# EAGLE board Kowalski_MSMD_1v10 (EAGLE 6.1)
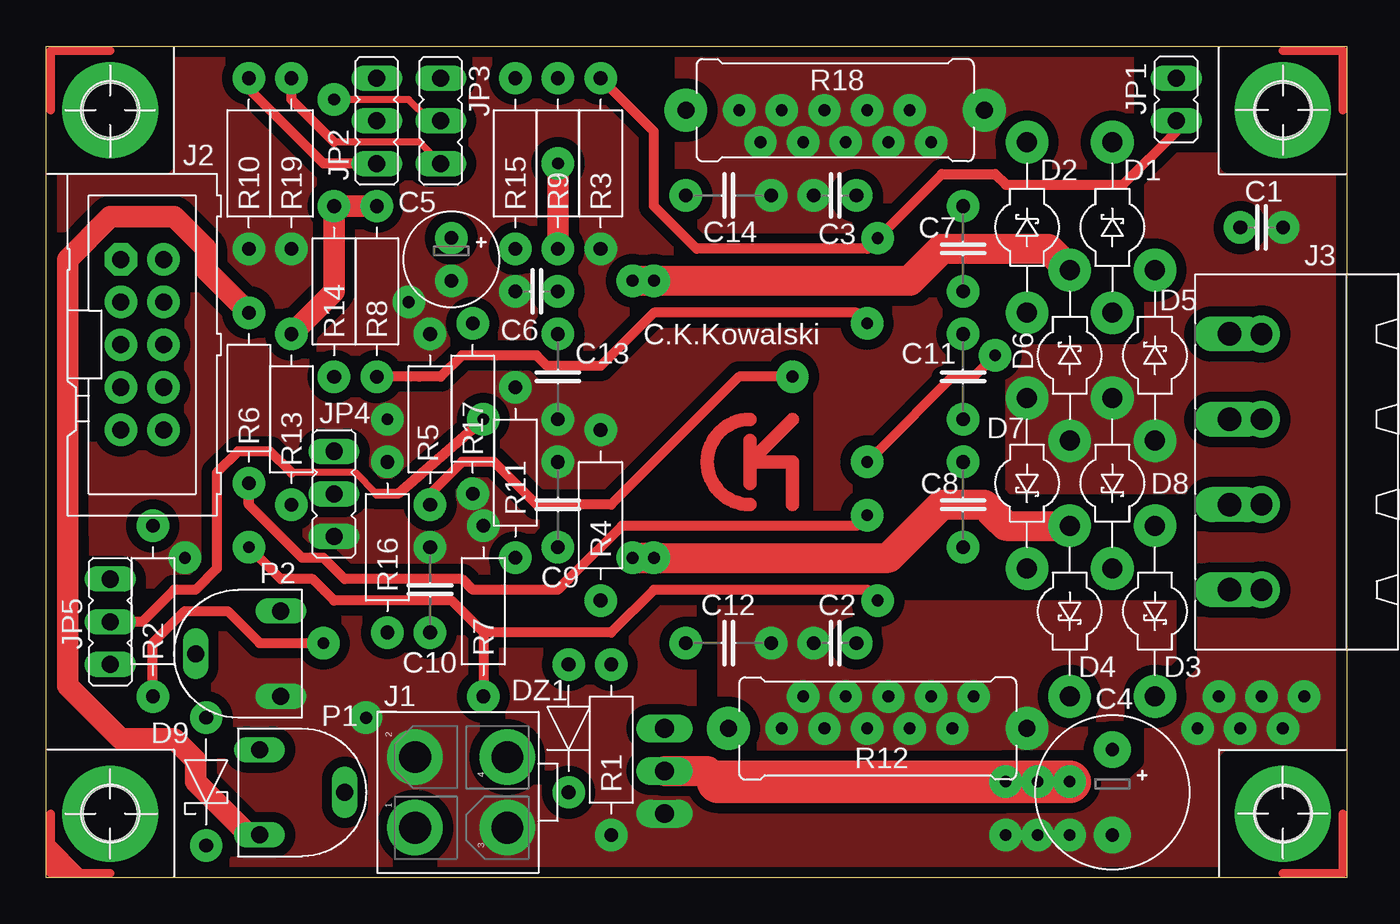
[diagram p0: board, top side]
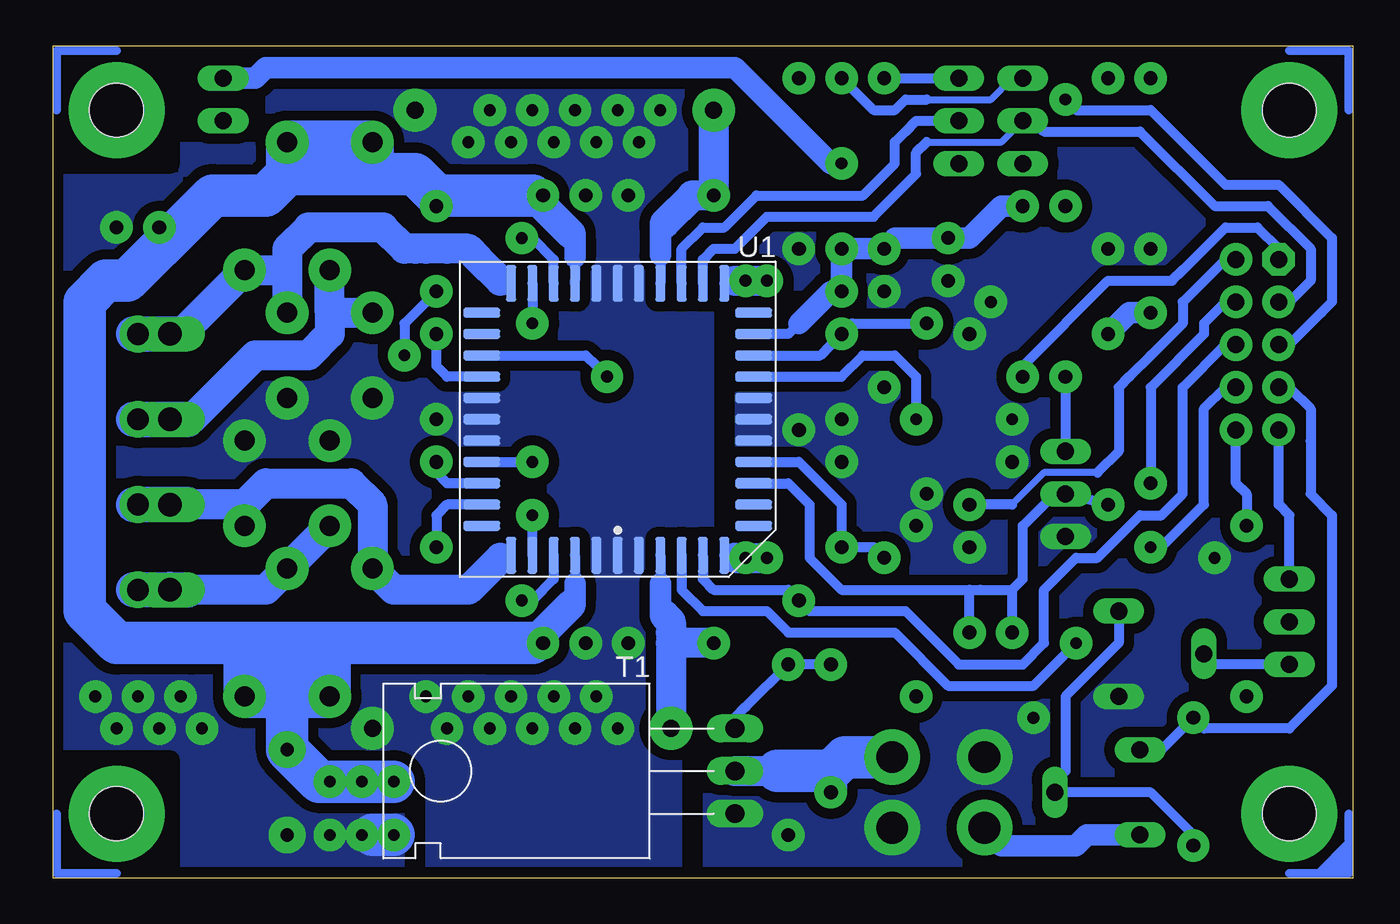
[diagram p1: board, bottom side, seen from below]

Size 77.47 x 49.53 mm. Coordinates in mm from the lower left corner, seen from the top.
Outline: 0,0 0,49.53 77.47,49.53 77.47,0 0,0
Copper layers (1*16): Top 0.035mm / dielectric 1.5mm / Bottom 0.035mm
Design rules: minimum track width 32mil, minimum drill 24mil, track to track 8mil, track to pad 8mil, pad to pad 8mil, via to via 8mil, smd to smd 8mil, copper to edge 25mil, drill to drill 8mil, minimum pad ring 10mil, minimum via ring 8mil, stop-mask expansion 4mil, vias tented up to drill 0mil, thermal gap 12mil
tRestrict: area 53.3,23.5 to 56.5,29.8; area 39.4,21.6 to 45.1,27.9; area 44.5,27.9 to 45.1,29.2; 21 lines
bRestrict: 6 lines

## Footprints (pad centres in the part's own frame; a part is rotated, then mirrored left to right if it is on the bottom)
C2.5 = drill 0.813 pad 1.93: 1 -1.27,0; 2 1.27,0
CE5 = drill 0.8 pad 2.184: + -2.54,0; - 2.54,0
CE2.5 = drill 0.8 pad 1.93: + -1.27,0; - 1.27,0
C5 = drill 0.813 pad 1.93: 1 -2.54,0; 2 2.54,0
DS = drill 1.194 pad 2.54: A 5.08,0; C -5.08,0
DS7,5 = drill 0.813 pad 1.93: A 3.81,0; C -3.81,0
DZ7,5 = drill 0.813 pad 1.93: A 3.81,0; C -3.81,0
MF-04-V = drill 1.9 pad 3.3: 1 2.1,-2.8; 2 -2.1,-2.8; 3 2.1,2.7; 4 -2.1,2.7
ML10 = drill 1.016 pad 1.93 octagon: 1 -5.08,-1.27 | drill 1.016 pad 1.93: 2 -5.08,1.27; 3 -2.54,-1.27; 4 -2.54,1.27; 5 0,-1.27; 6 0,1.27; 7 2.54,-1.27; 8 2.54,1.27; 9 5.08,-1.27; 10 5.08,1.27
MSTBA4 = drill 1.397 long: 1 -7.62,5.08; 2 -2.54,5.08; 3 2.54,5.08; 4 7.62,5.08
JP1 = drill 1.016 pad 1.422 long: 1 0,-1.27; 2 0,1.27
JP2 = drill 1.016 pad 1.422 long: 1 -2.54,0; 2 0,0; 3 2.54,0
CA6V = drill 1.016 long: A -2.54,-2.54; E 2.54,-2.54; S 0,2.54
0309/10 = drill 0.813 pad 1.93: 1 -5.08,0; 2 5.08,0
0617/17 = drill 1.016 pad 2.54: 1 -8.89,0; 2 8.89,0
TO220AH = drill 1.118 long: B 2.54,-6.35; C 0,-6.35; E -2.54,-6.35
STEPPER_PLCC44 = smd 0.6 x 2.2: 1 0,8.1; 2 -1.27,8.1; 3 -2.54,8.1; 4 -3.81,8.1; 5 -5.08,8.1; 6 -6.35,8.1; 18 -6.35,-8.1; 19 -5.08,-8.1; 20 -3.81,-8.1; 21 -2.54,-8.1; 22 -1.27,-8.1; 23 0,-8.1; 24 1.27,-8.1; 25 2.54,-8.1; 26 3.81,-8.1; 27 5.08,-8.1; 28 6.35,-8.1; 40 6.35,8.1; 41 5.08,8.1; 42 3.81,8.1; 43 2.54,8.1; 44 1.27,8.1 | smd 2.2 x 0.6: 7 -8.1,6.35; 8 -8.1,5.08; 9 -8.1,3.81; 10 -8.1,2.54; 11 -8.1,1.27; 12 -8.1,0; 13 -8.1,-1.27; 14 -8.1,-2.54; 15 -8.1,-3.81; 16 -8.1,-5.08; 17 -8.1,-6.35; 29 8.1,-6.35; 30 8.1,-5.08; 31 8.1,-3.81; 32 8.1,-2.54; 33 8.1,-1.27; 34 8.1,0; 35 8.1,1.27; 36 8.1,2.54; 37 8.1,3.81; 38 8.1,5.08; 39 8.1,6.35
CORNER_HOLE_3.2MM = hole 3.2: 0,0
CORNER_HOLE_3.2MM_SIGN = hole 3.2: 0,0

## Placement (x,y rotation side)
C1  100n  [C2.5]  72.39,38.73 0 top
C2  100n  [C2.5]  46.99,13.97 180 top
C3  3x100n  [C2.5]  46.99,40.64 180 top
C4  470u  [CE5]  63.5,5.08 270 top
C5  100u  [CE2.5]  24.13,36.83 270 top
C6  100n  [C2.5]  29.21,34.92 180 top
C7  220n  [C5]  54.61,37.47 270 top
C8  220n  [C5]  54.61,22.23 270 top
C9  1n  [C5]  30.48,22.23 90 top
C10  100n  [C5]  22.86,17.14 90 top
C11  220n  [C5]  54.61,29.84 270 top
C12  100n  [C5]  40.64,13.97 0 top
C13  1n  [C5]  30.48,29.84 90 top
C14  100n  [C5]  40.64,40.64 0 top
D1  DS  [DS]  63.5,38.73 270 top
D2  DS  [DS]  58.42,38.73 270 top
D3  8xBYV27  [DS]  66.04,15.88 90 top
D4  DS  [DS]  60.96,15.88 90 top
D5  DS  [DS]  66.04,31.11 270 top
D6  DS  [DS]  60.96,31.11 270 top
D7  DS  [DS]  58.42,23.5 90 top
D8  DS  [DS]  63.5,23.5 90 top
D9  BAT85  [DS7,5]  9.53,5.71 90 top
DZ1  30V  [DZ7,5]  31.11,8.89 90 top
J1  MF-04  [MF-04-V]  24.77,5.08 270 top
J2  ML10  [ML10]  5.71,31.75 270 top
J3  MSTBA4  [MSTBA4]  75.56,24.77 90 top
JP1  [JP1]  67.31,46.35 180 top
JP2  [JP2]  19.68,45.09 270 top
JP3  [JP2]  23.5,45.09 270 top
JP4  [JP2]  17.14,22.86 270 top
JP5  [JP2]  3.81,15.24 90 top
P1  4k7  [CA6V]  15.24,5.08 270 top
P2  4k7  [CA6V]  11.43,13.34 90 top
R1  4k7  [0309/10]  33.66,7.62 270 top
R2  4k7  [0309/10]  6.35,15.88 270 top
R3  4k7  [0309/10]  33.02,42.55 90 top
R4  4k7  [0309/10]  33.02,21.59 270 top
R5  4k7  [0309/10]  22.86,27.3 270 top
R6  15k  [0309/10]  12.06,28.57 270 top
R7  15k  [0309/10]  26.04,15.88 270 top
R8  15k  [0309/10]  19.68,34.92 270 top
R9  4k7  [0309/10]  30.48,42.55 90 top
R10  4k7  [0309/10]  12.06,42.55 90 top
R11  47k  [0309/10]  27.94,24.13 270 top
R12  0R22  [0617/17]  49.53,8.89 180 top
R13  10k  [0309/10]  14.61,27.3 90 top
R14  4k7  [0309/10]  17.14,34.92 270 top
R15  4k7  [0309/10]  27.94,42.55 90 top
R16  1k  [0309/10]  20.32,19.68 270 top
R17  47k  [0309/10]  25.4,27.94 90 top
R18  0R22  [0617/17]  46.99,45.72 180 top
R19  4k7  [0309/10]  14.61,42.55 90 top
T1  TIP130  [TO220AH]  43.18,6.35 90 bottom
U1  A3977  [STEPPER_PLCC44]  43.81,27.3 180 bottom
U$7  [CORNER_HOLE_3.2MM]  73.66,3.81 180 top
U$8  [CORNER_HOLE_3.2MM]  3.81,45.72 0 top
U$9  [CORNER_HOLE_3.2MM]  73.66,45.72 270 top
U$10  [CORNER_HOLE_3.2MM_SIGN]  3.81,3.81 90 top

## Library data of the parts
C1-C14 D1-D9 R1-R11 R13-R17 R19 U$7-U$10 = Std
DZ1 J1 R12 R18 = STANDARD_CK
J2 = con-ml; OC_FARNELL: unknown; OC_NEWARK: unknown
J3 = con-phoenix-508; MF: FARNELL; MPN: 1757268; OC_FARNELL: 3705195; OC_NEWARK: 71C4163
JP1-JP5 = jumper
P1 P2 = pot
T1 = MSMD_1v4
U1 = MSMD_1v1

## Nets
+5V: C5.+ C6.1 J1.1 JP1.1 P1.E R6.1 R8.1 R9.1 R13.2 R14.1 R15.1 U1.16
\!ENABLE: J2.4 R6.2 U1.41
\!HOME: R2.2 U1.4
\!HOME1: J2.10 R2.1
\!RESET: J2.1 R8.2 U1.27
\!SLEEP: J2.8 R7.2 U1.42
BOOST: D9.A J2.7 P1.A
CP1: C8.1 U1.37
CP2: C8.2 U1.38
DIR: J2.6 R4.2 U1.5
EXVREF: J2.9 JP5.3
GND: C1.2 C2.2 C3.2 C4.- C5.- C6.2 C9.2 C10.2 C11.2 C12.2 C13.1 C14.2 D5.A D6.A D7.A D8.A J1.2 J1.3 JP4.3 P2.A R1.2 R3.1 R4.1 R5.1 R7.1 R10.1 R11.1 R12.1 R16.1 R17.1 R18.1 R19.1 T1.E U1.1 U1.2 U1.11 U1.12 U1.13 U1.22 U1.23 U1.24 U1.33 U1.34 U1.35 U1.44
MS1: J2.5 JP3.2 U1.20
MS2: J2.3 JP2.2 U1.19
N$3: D9.C P1.S P2.E
N$4: C12.1 R12.2 U1.3
N$5: JP5.1 P2.S
N$6: JP2.1 R9.2
N$8: C14.1 R18.2 U1.21
N$9: JP4.1 R14.2
N$10: JP2.3 R10.2
N$12: JP3.3 R19.2
N$13: JP3.1 R15.2
N$14: DZ1.A R1.1 T1.B
OUT1A: D4.A D8.C J3.1 U1.6
OUT1B: D3.A D7.C J3.2 U1.40
OUT2A: D2.A D6.C J3.3 U1.18
OUT2B: D1.A D5.C J3.4 U1.28
PFD: C10.1 JP4.2 R13.1 R16.2 U1.9
RC1: C9.1 R11.2 U1.10
RC2: C13.2 R17.2 U1.15
SR: JP1.2 R3.2 U1.26
STEP: J2.2 R5.2 U1.31
VCC: C1.1 C2.1 C3.1 C4.+ C7.1 D1.C D2.C D3.C D4.C DZ1.C J1.4 T1.C U1.25 U1.43
VCP: C7.2 U1.36
VREF: JP5.2 U1.14
VREG: C11.1 U1.32

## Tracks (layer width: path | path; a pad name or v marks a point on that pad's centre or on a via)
+5V  (via drill 0.7 pad 1.93)
  Top 1.27: R8.1 R14.1 17.14,34.92 R13.2 | R6.1 9.53,36.2 9.53,37.47 7.62,39.37 3.81,39.37 1.27,36.83 1.27,20.32 1.27,11.43 3.17,9.53 4.45,8.26 7.62,8.26 8.89,6.99 8.89,5.71 12.06,2.54 P1.E | v30.48,42.55 30.48,41.91 R9.1
  Bottom 0.61: U1.16 33.66,32.38 33.02,33.02
  Bottom 1.27: R8.1 20.95,40.01 22.86,38.1 C5.+ 27.3,38.1 R15.1 R9.1 C6.1 31.11,34.92 33.02,33.02 | R6.1 13.34,33.66 R13.2 | JP1.1 65.41,47.62 64.77,48.26 36.83,48.26 34.29,45.72 31.11,42.55 v30.48,42.55 | J1.1 21.96,2.92 20.95,1.91 16.51,1.91 15.88,2.54 P1.E
\!ENABLE  (via drill 0.7 pad 1.93)
  Top 0.61: v48.9,21.59 48.26,20.95 34.29,20.95 31.11,17.78 30.48,17.14 25.4,17.14 24.77,17.78 17.78,17.78 16.51,19.05 15.24,19.05 12.06,22.23 | 12.06,22.23 R6.2 12.06,22.23
  Bottom 0.61: U1.41 v48.9,21.59 | R6.2 12.06,29.21 8.89,32.38 8.89,33.02 7.62,34.29 J2.4
\!HOME  (via drill 0.7 pad 1.93)
  Top 0.61: R2.2 6.35,13.97 8.26,15.88 10.79,15.88 12.7,13.97 v16.51,13.97
  Bottom 0.61: U1.4 40.01,17.14 38.73,15.88 34.92,15.88 33.66,14.61 28.57,14.61 27.3,14.61 24.13,11.43 19.05,11.43 17.14,13.34 v16.51,13.97
\!HOME1
  Bottom 0.61: R2.1 6.35,22.86 6.99,23.5 J2.10
\!RESET  (via drill 0.7 pad 1.93)
  Top 0.61: v48.9,33.02 48.26,33.66 36.2,33.66 35.56,33.02 33.02,30.48 29.84,30.48 29.21,31.11 24.77,31.11 23.5,29.84 22.23,29.84 R8.2
  Bottom 0.61: U1.27 v48.9,33.02 | R8.2 19.68,30.48 14.61,35.56 10.79,35.56 10.16,36.2 7.62,38.73 5.71,38.73 4.45,37.47 J2.1
\!SLEEP  (via drill 0.7 pad 1.93)
  Top 0.61: v49.53,16.51 48.9,17.14 36.2,17.14 33.66,14.61 26.04,14.61 | 26.04,14.61 24.13,16.51 17.14,16.51 15.88,17.78 13.97,17.78 v12.06,19.68 | 26.04,14.61 R7.2
  Bottom 0.61: U1.42 47.62,17.78 48.9,16.51 v49.53,16.51 | v12.06,19.68 11.43,19.68 8.89,22.23 8.89,27.94 7.62,29.21 J2.8
BOOST
  Bottom 0.61: P1.A 11.43,7.62 D9.A 8.89,8.89 3.81,8.89 1.27,11.43 1.27,21.59 2.54,22.86 2.54,26.04 2.54,27.94 3.81,29.21 J2.7
CP1
  Bottom 0.61: U1.37 53.98,23.5 54.61,24.13 C8.1
CP2
  Bottom 0.61: U1.38 53.98,22.23 54.61,21.59 C8.2
DIR
  Bottom 0.61: U1.5 38.73,17.78 38.1,17.14 33.66,17.14 R4.2 32.38,15.88 26.67,15.88 23.5,12.7 19.68,12.7 18.41,13.97 18.41,17.14 16.51,19.05 15.24,19.05 12.7,21.59 11.43,21.59 10.16,22.86 10.16,29.21 7.62,31.75 J2.6
EXVREF
  Bottom 0.61: JP5.3 3.81,21.59 4.45,22.23 J2.9
GND  (via drill 0.7 pad 1.93)
  Bottom 2.54: v57.15,2.54 58.42,2.54
  other vias: 21.59,34.29 20.32,27.3 74.93,10.79 72.39,10.79 69.85,10.79 19.05,9.53 8.26,19.05 43.81,8.89 46.35,8.89 48.9,8.89 51.44,8.89 53.98,8.89 52.7,10.79 55.24,10.79 50.16,10.79 47.62,10.79 45.09,10.79 41.27,45.72 43.81,45.72 46.35,45.72 48.9,45.72 51.44,45.72 42.55,43.81 45.09,43.81 47.62,43.81 50.16,43.81 52.7,43.81 59.05,2.54 60.96,2.54 71.12,8.89 73.66,8.89 68.58,8.89
  pour Bottom (isolate 0.61, no thermals): 76.83,48.9 76.83,0.64 0.64,0.64 0.64,48.9
  pour Top (isolate 0.61, no thermals): 76.83,48.9 76.83,0.64 0.64,0.64 0.64,48.9
MS1  (via drill 0.7 pad 1.93)
  Top 0.406: 22.86,45.09 21.59,46.35 v17.14,46.35
  Top 0.61: JP3.2 22.86,45.09
  Bottom 0.61: U1.20 40.01,37.47 38.73,38.73 37.47,38.73 35.56,40.64 29.21,40.64 27.3,42.55 27.3,43.81 26.67,44.45 26.04,45.09 JP3.2 | v17.14,46.35 16.51,45.72 12.06,45.72 7.62,41.27 4.45,41.27 1.27,38.1 1.27,34.29 1.91,33.66 3.81,31.75 J2.5
MS2
  Bottom 0.406: 25.4,43.81 20.95,43.81 JP2.2
  Bottom 0.61: U1.19 38.73,36.83 38.1,37.47 36.83,37.47 34.92,39.37 31.11,39.37 28.57,39.37 26.04,41.91 26.04,43.18 25.4,43.81 | JP2.2 19.05,45.09 18.41,44.45 12.7,44.45 8.26,40.01 5.08,40.01 2.54,37.47 2.54,35.56 3.81,34.29 J2.3
N$1  (via drill 3.2 pad 5.71)
  other vias: 73.66,45.72
N$2  (via drill 3.2 pad 5.71)
  other vias: 73.66,3.81
N$3
  Bottom 0.61: D9.C 9.53,2.54 12.06,5.08 P1.S 17.78,5.71 17.14,6.35 17.14,10.79 13.97,13.97 P2.E
N$4
  Bottom 0.61: U1.3 41.27,17.53
  Bottom 1.27: 41.02,15.62 41.27,15.88 41.27,17.53
  Bottom 1.778: C12.1 40.64,13.97 | 40.64,13.97 R12.2 | 40.64,13.97 40.64,14.61 40.64,15.24 41.02,15.62
N$5
  Bottom 0.61: JP5.1 8.89,12.7 P2.S
N$6
  Bottom 0.406: 25.4,46.35 21.59,46.35 20.32,47.62
  Bottom 0.61: R9.2 28.57,45.72 27.3,45.72 26.67,46.35 25.4,46.35 | 20.32,47.62 JP2.1
N$7  (via drill 3.2 pad 5.71)
  other vias: 3.81,45.72
N$8
  Bottom 0.61: 41.27,37.08 U1.21
  Bottom 1.27: 41.02,38.99 41.27,38.73 41.27,37.08
  Bottom 1.778: 41.02,38.99 39.37,40.64 C14.1 38.1,41.91 R18.2
N$9
  Bottom 0.61: R14.2 JP4.1
N$10
  Top 0.61: JP2.3 16.51,42.55 12.06,46.99 R10.2
N$11  (via drill 3.2 pad 5.71)
  other vias: 3.81,3.81
N$12
  Top 0.406: JP3.3 22.23,43.81 17.14,43.81
  Top 0.61: 17.14,43.81 14.61,46.35 R19.2
N$13
  Bottom 0.61: R15.2 JP3.1
N$14
  Bottom 0.61: DZ1.A R1.1 36.2,10.16 36.83,9.53 T1.B
N$15
  Top 0.813: 41.91,26.04 41.91,24.77 | 41.91,24.77 41.91,23.5 | 41.91,24.77 44.45,27.3 | 41.91,24.77 44.45,24.77 44.45,22.23
N$16
  Top 0.813: 41.91,27.3 arc180 41.91,22.23
OUT1A  (via drill 0.7 pad 1.93, 1.3 pad 2.18)
  Top 1.778: v34.92,19.05 35.56,19.05 v36.2,19.05 50.16,19.05 53.34,22.23 55.88,22.23 56.52,21.59 57.15,20.95 D4.A
  Bottom 0.61: U1.6 37.31,19.05 36.83,19.05
  Bottom 1.778: 36.83,19.05 v34.92,19.05 | D4.A D8.C 64.14,17.78 64.77,17.14 69.47,17.14
  Bottom 2.083: 70.51,17.14 v72.39,17.14 | v72.39,17.14 72.64,17.14 v72.39,17.14
  Bottom 2.108: 69.47,17.14 J3.1 70.51,17.14 70.51,17.17
OUT1B  (via drill 1.3 pad 2.18)
  Bottom 0.61: U1.40 50.32,19.05 50.8,19.05
  Bottom 1.778: 50.8,19.05 52.7,17.14 53.34,17.14 55.24,17.14 57.15,17.14 D7.C 58.42,22.23 59.69,23.5 64.77,23.5 66.04,22.23 | D3.A 66.04,22.23 | 66.04,22.23 69.47,22.23
  Bottom 2.083: v72.39,22.23 72.64,22.23 v72.39,22.23
  Bottom 2.108: 69.47,22.23 J3.2 | J3.2 v72.39,22.23 J3.2
OUT2A  (via drill 0.7 pad 1.93, 1.3 pad 2.18)
  Top 1.778: v34.92,35.56 35.56,35.56 48.26,35.56 48.9,35.56 51.44,35.56 53.34,37.47 59.69,37.47 D6.C
  Bottom 0.61: U1.18 37.31,35.56 36.83,35.56
  Bottom 1.27: 71.78,27.33 71.75,27.3 v72.39,27.3
  Bottom 1.778: 36.83,35.56 v36.2,35.56 | v36.2,35.56 35.56,35.56 | 35.56,35.56 v34.92,35.56 | 60.96,33.66 60.96,32.38 62.23,31.11 65.41,31.11 69.22,27.3 69.47,27.3 | 60.96,33.66 D2.A | 60.96,33.66 D6.C | v36.2,35.56 35.56,35.56
  Bottom 2.083: 71.75,27.3 v72.39,27.3 | v72.39,27.3 72.64,27.3 v72.39,27.3
  Bottom 2.108: 69.85,27.3 69.47,27.3 69.85,27.3 | 69.85,27.3 J3.3 | J3.3 71.75,27.3 | v72.39,27.3 J3.3 | J3.3 69.85,27.3 | 69.85,27.3 J3.3 | 69.85,27.3 J3.3
OUT2B  (via drill 1.3 pad 2.18)
  Bottom 0.61: U1.28 50.32,35.56 50.8,35.56
  Bottom 1.27: 71.78,32.36 71.75,32.38
  Bottom 1.778: 50.8,35.56 52.07,36.83 52.7,37.47 53.98,37.47 55.24,37.47 55.88,37.47 56.52,37.47 57.78,38.73 62.23,38.73 63.5,37.47 63.5,36.2 | 63.5,36.2 D1.A | 63.5,36.2 D5.C 69.85,32.38
  Bottom 2.083: 71.75,32.38 v72.39,32.38 | v72.39,32.38 72.64,32.38 v72.39,32.38
  Bottom 2.108: v72.39,32.38 J3.4 69.85,32.38
PFD
  Bottom 0.61: U1.9 33.66,23.5 32.38,22.23 32.38,19.05 30.48,17.14 22.86,17.14 | 22.86,17.14 22.23,17.14 20.32,17.14 | 20.32,17.14 R16.2 | 20.32,17.14 19.68,17.78 19.68,20.95 17.78,22.86 JP4.2 R13.1 | C10.1 22.86,17.14
RC1
  Bottom 0.61: U1.10 33.02,24.77 32.38,24.13 30.48,22.23 C9.1 28.57,19.68 R11.2
RC2
  Bottom 0.61: U1.15 31.75,31.11 31.11,31.75 C13.2 29.84,33.02 R17.2
SR  (via drill 0.7 pad 1.93)
  Top 0.61: R3.2 36.2,44.45 36.2,40.01 38.73,37.47 48.9,37.47 v49.53,38.1 53.34,41.91 56.52,41.91 57.15,41.27 64.14,41.27 67.31,44.45 JP1.2
  Bottom 0.61: U1.26 47.62,36.83 48.9,38.1 v49.53,38.1
STEP  (via drill 0.7 pad 1.93)
  Top 0.61: v44.45,29.84 43.81,29.84 41.27,29.84 33.66,22.23 29.21,22.23 26.67,24.77 24.77,24.77 22.86,22.86 R5.2
  Bottom 0.406: 15.24,24.13 18.41,24.13 20.32,22.23
  Bottom 0.61: U1.31 45.72,31.11 45.09,30.48 v44.45,29.84 | 20.32,22.23 R5.2 | 15.24,24.13 13.97,25.4 13.97,29.21 13.34,29.84 12.06,31.11 10.16,33.02 10.16,34.29 7.62,36.83 J2.2
VCC  (via drill 0.7 pad 1.93)
  Top 1.778: T1.C 39.37,6.35 40.01,5.71
  Top 2.54: 40.01,5.71 v57.15,5.71 v60.96,5.71
  Bottom 0.61: U1.43 46.35,17.53 | 46.35,36.96 46.35,35.56 U1.25
  Bottom 1.016: 48.9,13.97 C2.1 48.26,14.61
  Bottom 1.27: 46.35,17.53 46.35,16.51 46.61,16.26 | 46.61,38.35 46.35,38.1 46.35,36.96 | 48.26,40.01 C3.1 48.9,40.64 | 69.85,38.73 C1.1
  Bottom 1.778: T1.C 34.29,6.35 | 46.61,16.26 48.26,14.61 | 48.26,40.01 46.61,38.35 | C7.1 54.61,40.64
  Bottom 1.93: DZ1.C 31.11,6.35
  Bottom 2.54: 34.29,6.35 31.11,6.35 30.29,7.18 J1.4 | v60.96,5.71 61.59,5.71 C4.+ 63.5,10.79 D4.C 60.96,13.97 | v60.96,5.71 v59.05,5.71 | v59.05,5.71 v57.15,5.71 | v59.05,5.71 v60.96,5.71 | 60.96,13.97 63.5,13.97 66.04,13.97 | 66.04,13.97 69.22,13.97 73.66,13.97 75.56,15.88 75.56,34.29 74.3,35.56 73.03,35.56 72.39,36.2 69.85,38.73 67.94,40.64 64.77,40.64 63.5,41.91 | 63.5,41.91 58.42,41.91 | D3.C 66.04,13.97 | D1.C 63.5,41.91 | D2.C 58.42,41.91 | 48.9,40.64 53.34,40.64 53.98,40.64 54.61,40.64 55.88,41.91 58.42,41.91 | 48.9,13.97 50.8,13.97 51.44,13.97 60.96,13.97
VCP  (via drill 0.7 pad 1.93)
  Top 0.61: v48.9,24.77 49.53,25.4 53.98,29.84 55.24,29.84 v56.52,31.11
  Bottom 0.61: U1.36 49.53,24.77 v48.9,24.77 | C7.2 56.52,33.02 v56.52,31.11
VREF  (via drill 0.7 pad 1.93)
  Top 0.406: 19.68,22.86 18.41,24.13 14.61,24.13
  Top 0.61: v26.04,27.3 20.95,22.86 19.68,22.86 | 14.61,24.13 13.34,25.4 11.43,25.4 10.16,24.13 10.16,18.41 8.89,17.14 7.62,17.14 5.71,15.24 JP5.2
  Bottom 0.61: U1.14 31.11,29.84 30.48,29.84 29.21,31.11 27.3,31.11 26.04,29.84 v26.04,27.3
VREG
  Bottom 0.61: U1.32 53.98,29.84 54.61,30.48 C11.1
(copper drawn outside any net)
  shapes: Bottom area x4

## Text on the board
tPlace: C.K.Kowalski
tValues: 100n | 100n | 100n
